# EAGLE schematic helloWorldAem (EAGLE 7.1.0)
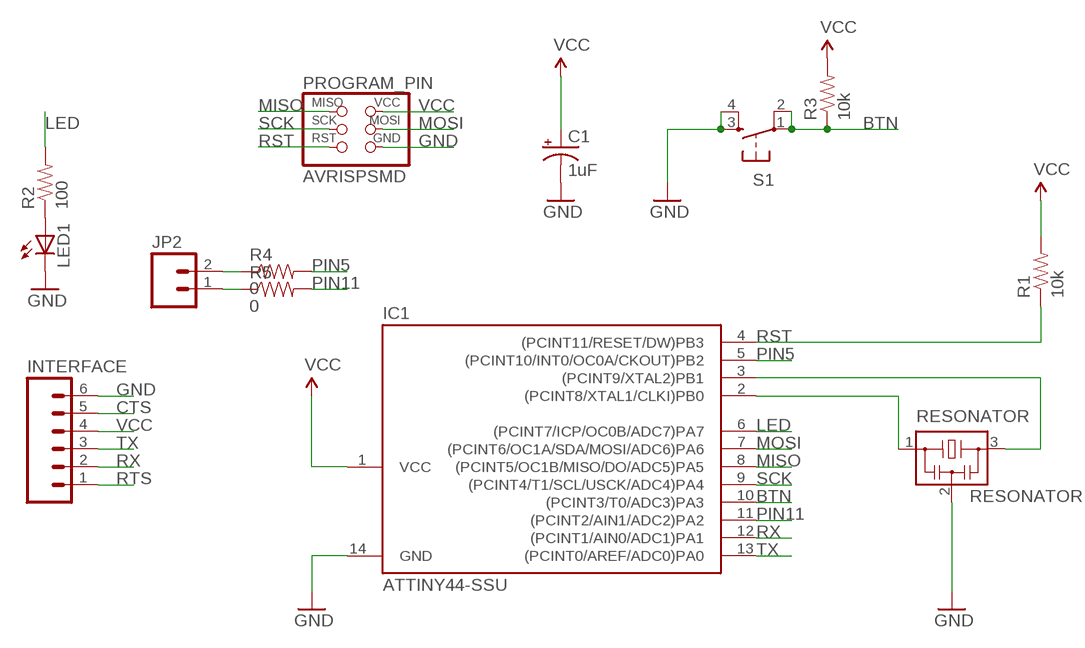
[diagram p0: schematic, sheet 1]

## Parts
C1  1uF  CAP_POL1206  [EIA3216]
IC1  ATTINY44-SSU  [SOIC14]
INTERFACE  M06SMD  [1X06-SMD]
JP2  M02  [1X02_LONGPADS]
LED1  LED1206  [LED-1206]
PROGRAM_PIN  AVRISPSMD  [2X03SMD]
R1  10k  RESISTOR1206  [1206]
R2  100  RESISTOR1206  [1206]
R3  10k  RESISTOR1206  [1206]
R4  0  RESISTOR1206  [1206]
R5  0  RESISTOR1206  [1206]
RESONATOR  RESONATOR  [EFOBM]
S1  6MM_SWITCH6MM_SWITCH  [6MM_SWITCH]

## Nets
BTN: IC1.10((PCINT3/T0/ADC3)PA3) R3.1 S1.1(P) S1.2(P1)
CTS: INTERFACE.5
GND: C1.C(-) IC1.14(GND) INTERFACE.6 LED1.C PROGRAM_PIN.6(GND) RESONATOR.2 S1.3(S) S1.4(S1)
LED: IC1.6((PCINT7/ICP/OC0B/ADC7)PA7) R2.2
MISO: IC1.8((PCINT5/OC1B/MISO/DO/ADC5)PA5) PROGRAM_PIN.1(MISO)
MOSI: IC1.7((PCINT6/OC1A/SDA/MOSI/ADC6)PA6) PROGRAM_PIN.4(MOSI)
N$1: JP2.2 R4.1
N$2: IC1.3((PCINT9/XTAL2)PB1) RESONATOR.3
N$3: IC1.2((PCINT8/XTAL1/CLKI)PB0) RESONATOR.1
N$4: LED1.A R2.1
N$5: JP2.1 R5.1
PIN5: IC1.5((PCINT10/INT0/OC0A/CKOUT)PB2) R4.2
PIN11: IC1.11((PCINT2/AIN1/ADC2)PA2) R5.2
RST: IC1.4((PCINT11/RESET/DW)PB3) PROGRAM_PIN.5(RST) R1.1
RTS: INTERFACE.1
RX: IC1.12((PCINT1/AIN0/ADC1)PA1) INTERFACE.2
SCK: IC1.9((PCINT4/T1/SCL/USCK/ADC4)PA4) PROGRAM_PIN.3(SCK)
TX: IC1.13((PCINT0/AREF/ADC0)PA0) INTERFACE.3
VCC: C1.A(+) IC1.1(VCC) INTERFACE.4 PROGRAM_PIN.2(VCC) R1.2 R3.2

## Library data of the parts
C1 = 01_SparkFun:CAP_POL: Capacitor Polarized
IC1 = fab:ATTINY44
INTERFACE = 01_SparkFun:M06: Header 6 Standard 6-pin 0.1" header. Use with straight break away headers (SKU : PRT-00116), right angle break away headers (PRT-00553), swiss pins (PRT-00743), machine pins (PRT-00117), and female headers (PRT-00115). Molex polarized connector foot print use with SKU : PRT-08094 with associated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
JP2 = 01_SparkFun:M02: Header 2
LED1 = 01_SparkFun:LED: LEDs
PROGRAM_PIN = fab:AVRISP
R1-R5 = 01_SparkFun:RESISTOR: Resistor
RESONATOR = fab:RESONATOR
S1 = fab:6MM_SWITCH: OMRON SWITCH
